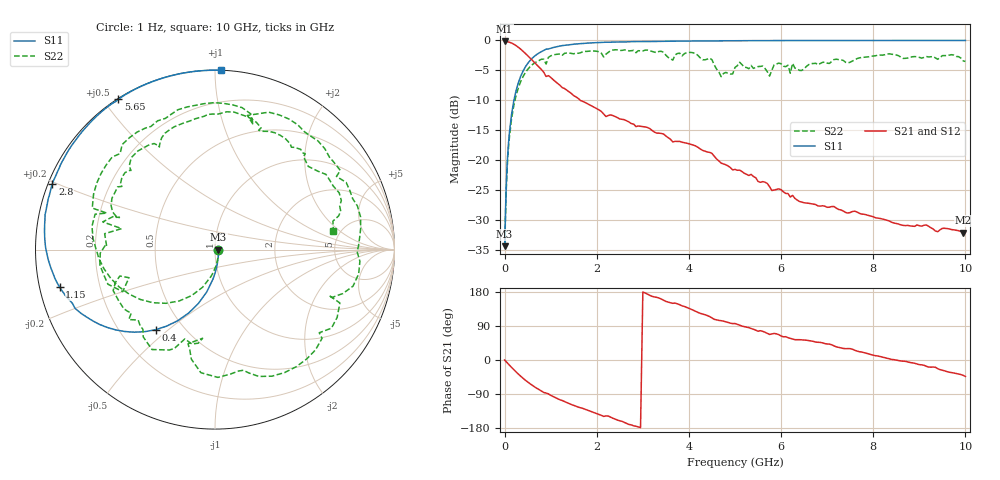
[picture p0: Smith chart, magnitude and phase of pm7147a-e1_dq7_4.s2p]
# GHz S DB R 50
! S-Parameters data
! Freq  dbS11  angS11  dbS21  angS21  dbS12  angS12  dbS22  angS22
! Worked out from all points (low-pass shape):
!   279 points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, 1 Hz to 10 GHz, reference 50 ohm
!   highest |S21| = -0.17 dB at 3.981 kHz (marker M1); lowest = -32.0 dB at 9.95 GHz (marker M2)
!   |S21| within 3 dB of the highest: start of sweep to 583 MHz
!   lowest |S11| = -34.3 dB at 1.995 kHz (marker M3), VSWR 1.04, Z = 52 - j0.000331 ohm
!   |S11| at or under -10 dB: start of sweep to 201.3 MHz
!   |S22| runs from -34.3 to -1.6 dB; largest |S21 - S12| = 0
!   S11 on the Smith chart (normalised r, x): 1 Hz: 1.04, -0.00; 400 MHz: 0.35, -0.45; 1.15 GHz: 0.06, -0.12; 2.8 GHz: 0.01, +0.19; 5.65 GHz: 0.00, +0.55; 10 GHz: 0.00, +1.03
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1e-09  -34.29 -0.0  -0.17 -0.0  -0.17 -0.0  -34.29 -0.0
1.9953e-06  -34.29 -0.0  -0.17 -0.0  -0.17 -0.0  -34.29 -0.0
3.9811e-06  -34.29 -0.0  -0.17 -0.0  -0.17 -0.0  -34.29 -0.0
0.03981072  -23.31 -77.5  -0.19 -5.2  -0.19 -5.2  -24.01 -78.1
0.1  -15.71 -93.8  -0.29 -13.1  -0.29 -13.1  -16.45 -98.3
0.4  -5.11 -126.5  -1.80 -48.2  -1.80 -48.2  -6.02 -146.2
0.75  -2.07 -149.7  -4.49 -78.2  -4.49 -78.2  -3.33 174.9
1.15  -1.01 -166.3  -7.15 -102.1  -7.15 -102.1  -2.29 142.1
1.7  -0.49 178.6  -10.18 -127.8  -10.18 -127.8  -1.87 104.8
2.3  -0.29 166.4  -12.41 -150.8  -12.41 -150.8  -1.70 68.7
2.8  -0.20 158.1  -13.94 -173.7  -13.94 -173.7  -1.66 32.3
3.35  -0.15 150.0  -15.46 163.4  -15.46 163.4  -1.83 -4.6
3.9  -0.11 142.7  -17.04 141.4  -17.04 141.4  -2.22 -39.6
4.15  -0.09 139.5  -17.61 128.2  -17.61 128.2  -2.23 -65.8
4.55  -0.07 134.7  -19.29 107.3  -19.29 107.3  -4.09 -102.2
5.05  -0.04 129.0  -21.64 94.1  -21.64 94.1  -4.22 -114.5
5.65  -0.04 122.7  -23.63 73.3  -23.63 73.3  -4.66 -161.7
6.7  -0.01 112.6  -27.28 49.2  -27.28 49.2  -3.85 150.3
8.35  -0.01 99.1  -30.11 3.0  -30.11 3.0  -2.23 82.2
9.35  -0.00 92.2  -31.77 -19.2  -31.77 -19.2  -2.91 46.4
9.95  -0.00 88.4  -32.02 -40.4  -32.02 -40.4  -3.40 13.6
10  -0.00 88.1  -31.95 -43.3  -31.95 -43.3  -3.51 9.1
